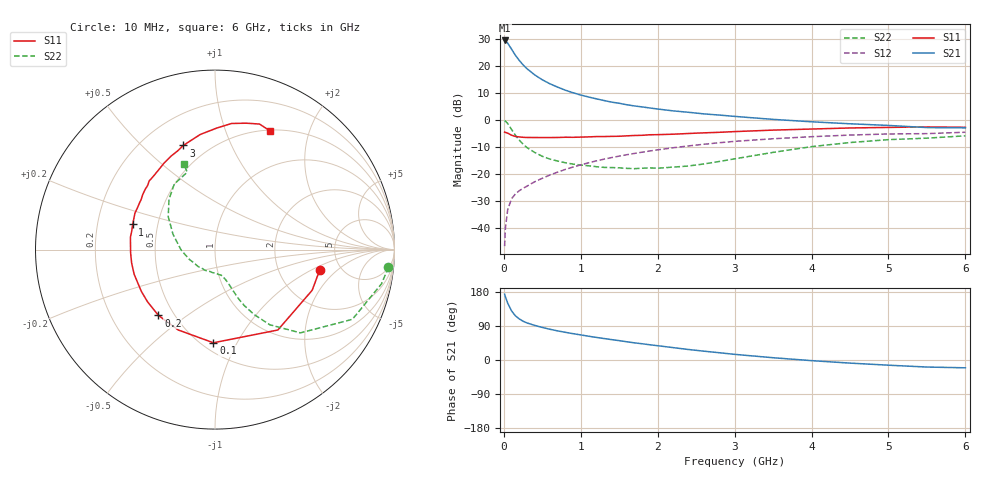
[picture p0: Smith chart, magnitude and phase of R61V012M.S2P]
! SIEMENS Small Signal Semiconductors
! BFR193
! Si NPN RF Bipolar Junction Transistor in SOT23
! VCE = 1 V  IC = 12 mA
! Common Emitter S-Parameters:  May  1996
# GHz  S  MA  R  50
!  f  S11  S21  S12  S22
! GHz  MAG  ANG  MAG  ANG  MAG  ANG  MAG  ANG
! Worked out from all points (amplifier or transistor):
!   36 points, 10 MHz to 6 GHz, reference 50 ohm
!   highest |S21| = 29.5 dB at 10 MHz (marker M1)
!   |S21| within 3 dB of that: start of sweep to 95.25 MHz
!   unconditionally stable (mu >= 1): 636 MHz to 2.165 GHz
!   at 250 MHz: K = 0.71, MSG = 23.0 dB, |S12| = -25.4 dB
!   at 1.4 GHz: K = 1.05, MAG = 9.0 dB, |S12| = -14.0 dB
!   at 6 GHz: K = 0.97, MSG = 0.8 dB, |S12| = -4.6 dB
!   S11 on the Smith chart (normalised r, x): 10 MHz: 3.44, -1.24; 100 MHz: 0.57, -0.81; 200 MHz: 0.41, -0.39; 1 GHz: 0.36, +0.13; 3 GHz: 0.37, +0.67; 6 GHz: 0.51, +1.44
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0.01  0.594 -11.3  30.01 173.6  0.0045 82.1  0.9713 -5.8
0.02  0.5869 -22.7  29.49 167.0  0.0096 82.8  0.9472 -11.6
0.05  0.5686 -52.0  26.71 150.1  0.0214 69.1  0.8585 -26.9
0.1  0.5192 -91.0  20.74 129.7  0.0342 59.2  0.6644 -44.3
0.15  0.4925 -114.7  15.96 116.7  0.042 54.9  0.5183 -53.9
0.2  0.4835 -130.7  12.81 108.5  0.0482 54.2  0.4228 -58.9
0.25  0.4752 -142.3  10.56 102.3  0.0535 54.8  0.3537 -62.3
0.3  0.4718 -150.5  8.977 97.9  0.0587 56.2  0.307 -64.3
0.4  0.4709 -163.0  6.891 91.3  0.0707 58.4  0.2489 -66.3
0.5  0.4705 -170.7  5.569 85.9  0.0823 60.2  0.2106 -67.9
0.6  0.4705 -177.9  4.69 81.1  0.0949 61.4  0.1871 -69.6
0.7  0.4716 176.6  4.062 76.8  0.1072 62.1  0.172 -71.3
0.8  0.4763 171.6  3.569 73.0  0.1202 62.0  0.1597 -73.3
1  0.4796 163.0  2.905 66.2  0.146 61.6  0.1451 -77.3
1.1  0.4839 159.1  2.672 62.8  0.1593 61.2  0.1407 -81.1
1.6  0.5062 142.7  1.913 48.0  0.2257 56.7  0.1257 -102.0
2.2  0.5426 125.8  1.473 32.7  0.3037 49.2  0.1327 -133.9
3  0.6068 106.9  1.163 14.9  0.3996 37.1  0.1892 -179.5
3.5  0.6467 97.3  1.024 6.0  0.4467 29.2  0.2493 159.9
4.5  0.7088 82.5  0.848 -8.2  0.5229 14.7  0.38 132.4
5.5  0.7422 70.5  0.721 -18.6  0.5562 0.4  0.4583 109.7
6  0.7288 65.0  0.713 -20.6  0.5907 -3.8  0.5063 110.1
